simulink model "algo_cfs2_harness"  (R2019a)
settings: configuration reference "configurationSettings" (kept in a data dictionary, not in this file)
undefined symbols (not defined in the file or in its folder): algo_cfs2_fp

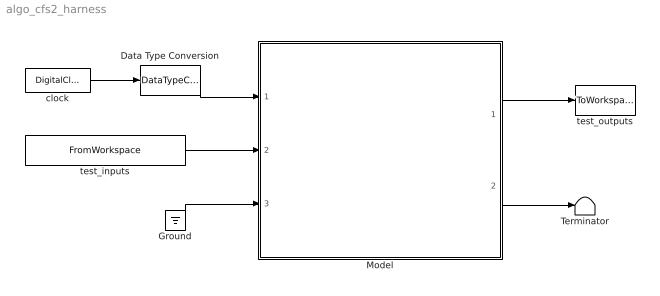
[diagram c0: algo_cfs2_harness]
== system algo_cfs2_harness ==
  Data Type Conversion : DataTypeConversion  OutDataTypeStr=single
  Ground : Ground
  Model : ModelReference  ModelNameDialog=algo_cfs2.slx  SimulationMode=Normal  ModelReferenceVersion=1.792  SimulationMode=Normal
  Terminator : Terminator
  clock : DigitalClock  SampleTime=algo_cfs2_fp.timing.dt
  test_inputs : FromWorkspace  VariableName=algo_cfs2_inbus1  OutDataTypeStr=Bus: algo_cfs2_inBus  SampleTime=algo_cfs2_fp.timing.dt  Interpolate=off  OutputAfterFinalValue=Holding final value
  test_outputs : ToWorkspace  VariableName=simout  SaveFormat=Timeseries  SampleTime=-1
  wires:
  Model/1 -> test_outputs/1
  clock/1 -> Data Type Conversion/1
  test_inputs/1 -> Model/2
  Data Type Conversion/1 -> Model/1
  Ground/1 -> Model/3
  Model/2 -> Terminator/1
